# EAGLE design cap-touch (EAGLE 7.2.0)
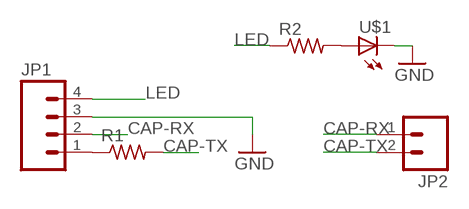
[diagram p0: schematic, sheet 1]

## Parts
JP1  M04LONGPADS  [1X04_LONGPADS]
JP2  M02  [1X02_LONGPADS]
R1  RES-US1206FAB  [R1206FAB]
R2  RES-US1206FAB  [R1206FAB]
U$1  LED1206  [1206]

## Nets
CAP-RX: JP1.2 JP2.1
CAP-TX: JP2.2 R1.2
GND: JP1.3 U$1.2(C)
LED: JP1.4 R2.1
N$1: JP1.1 R1.1
N$3: R2.2 U$1.1(A)

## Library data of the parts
JP1 = 01_SparkFun:M04: Header 4 Standard 4-pin 0.1" header. Use with straight break away headers (SKU : PRT-00116), right angle break away headers (PRT-00553), swiss pins (PRT-00743), machine pins (PRT-00117), and female headers (PRT-00115). Molex polarized connector foot print use with SKU : PRT-08231 with associated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
JP2 = 01_SparkFun:M02: Header 2
R1 R2 = 01fab:RES-US: Resistor (US Symbol)
U$1 = 01_FAB_Hello:LED

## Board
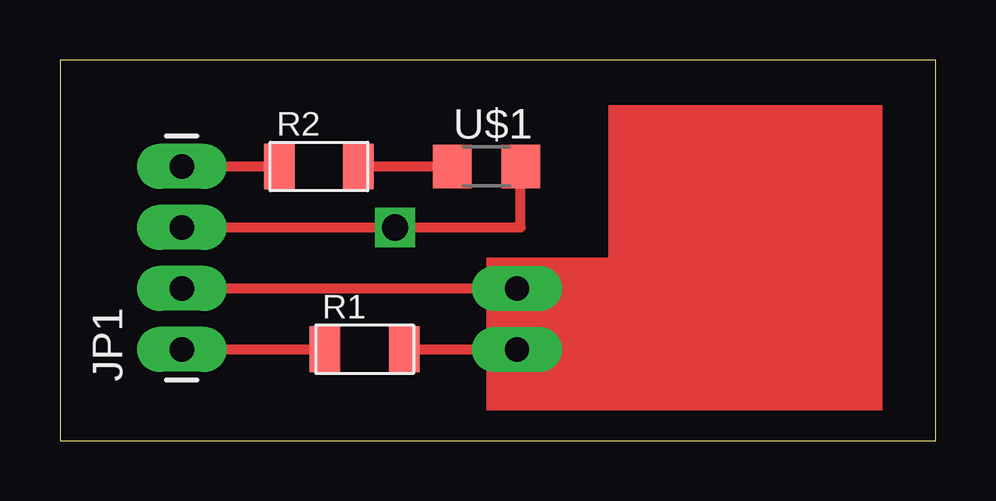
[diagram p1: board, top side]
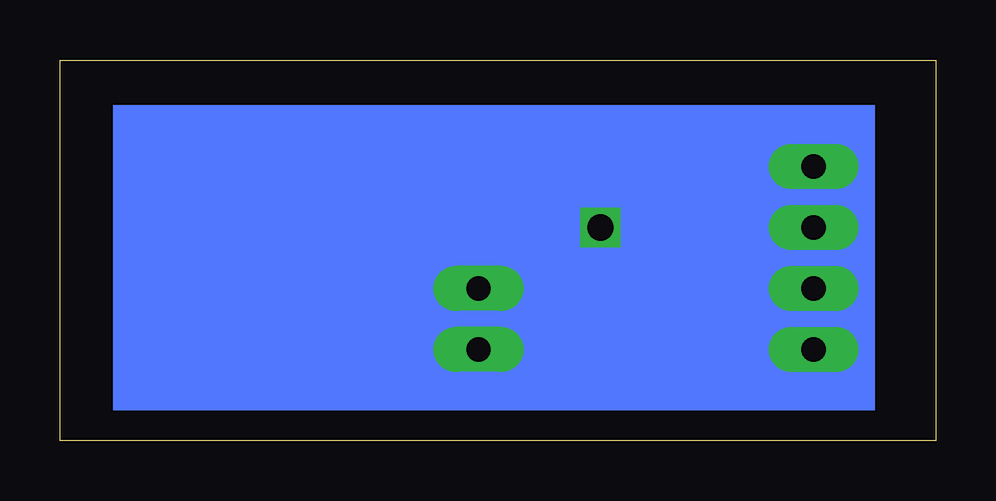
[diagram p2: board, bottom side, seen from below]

Size 36.5 x 15.87 mm. Coordinates in mm from the lower left corner, seen from the top.
Outline: 0,0 36.5,0 36.5,15.87 0,15.87 0,0
Copper layers (1*16): Top 0.035mm / dielectric 1.5mm / Bottom 0.035mm
Design rules "default": minimum track width 10mil, minimum drill 24mil, track to track 8mil, track to pad 8mil, pad to pad 8mil, via to via 8mil, smd to smd 8mil, copper to edge 40mil, drill to drill 8mil, minimum pad ring 10mil, minimum via ring 8mil, stop-mask expansion 4mil, vias tented up to drill 0mil, thermal gap 10mil

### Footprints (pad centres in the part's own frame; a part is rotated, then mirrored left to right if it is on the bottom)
1X04_LONGPADS = drill 1.016 pad 1.88 long: 1 0,0; 2 2.54,0; 3 5.08,0; 4 7.62,0
1X02_LONGPADS = drill 1.016 pad 1.88 long: 1 0,0; 2 2.54,0
R1206FAB = smd 1.27 x 1.905: 1 -1.651,0; 2 1.651,0
1206 = smd 1.6 x 1.803: 1 -1.422,0; 2 1.422,0

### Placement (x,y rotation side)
JP1  5.08,3.81 90 top
JP2  19.05,6.35 270 top
R1  12.7,3.81 0 top
R2  10.79,11.43 0 top
U$1  17.78,11.43 0 top

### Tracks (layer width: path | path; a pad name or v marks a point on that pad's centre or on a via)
CAP-RX
  Top 0.406: JP1.2 JP2.1 20.32,6.35
CAP-TX
  Top 0.406: R1.2 JP2.2
GND  (via drill 1.1)
  Top 0.406: JP1.3 v13.97,8.89 19.2,8.89 U$1.2
LED
  Top 0.406: JP1.4 R2.1
N$1
  Top 0.406: JP1.1 R1.1
N$3
  Top 0.406: R2.2 U$1.1
(copper drawn outside any net)
  shapes: Bottom area x1, Top area x4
